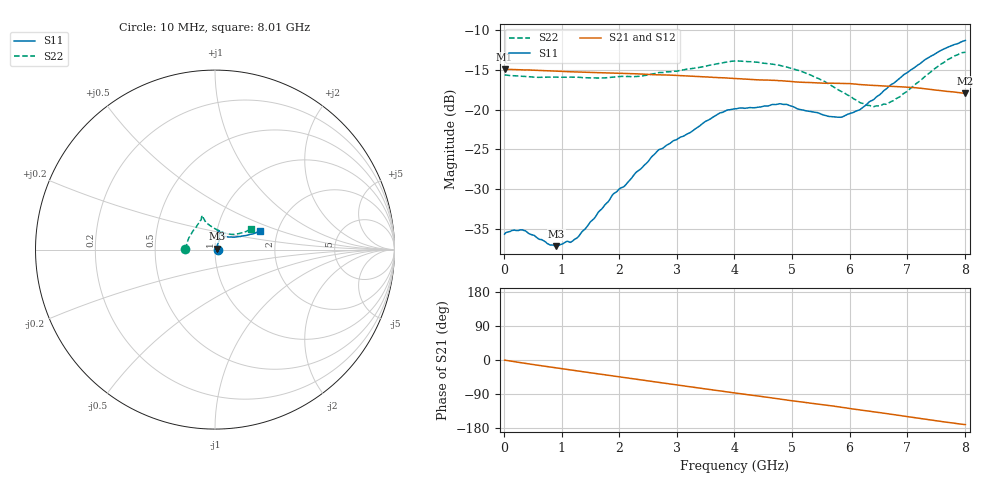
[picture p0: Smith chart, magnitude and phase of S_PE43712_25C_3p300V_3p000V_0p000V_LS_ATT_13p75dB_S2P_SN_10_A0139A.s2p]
! DEVICE ID: PE43712
! File Path: z:\PE43713\PE43713_CHAR_NOM_04292014\AMB\3p300\LS_ATT_13p75dB\PE43713_AMB_3p300V_3p000V_0p000V_LS_ATT_13p75dB_S2P_SN_10_A0139A.s2p
! Serial: 10
! Lot: A0139A
! Temp: 25C
! VDD: 3.300
! VSS: 0.000
! Control_Hi: 3.000
! Control_Lo: 0.000
! Attenuation Step: 13.75dB
! Port 1: RF1
! Port 2: RF2
! ThroughPath:1-2
! IDD: 0.0001471566
! ISS: -7.97e-008
#  Hz  S  RI  R  50
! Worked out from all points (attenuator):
!   801 points, 10 MHz to 8.01 GHz, reference 50 ohm
!   highest |S21| = -14.95 dB at 10 MHz (marker M1); lowest = -18.0 dB at 8.01 GHz (marker M2)
!   lowest |S11| = -37.2 dB at 910 MHz (marker M3), VSWR 1.03, Z = 51.3 + j0.588 ohm
!   |S11| at or under -10 dB: start of sweep to end of sweep
!   |S22| runs from -19.6 to -12.8 dB; largest |S21 - S12| = 0.00065
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1e7  0.0165 0.000311  0.1788 -0.00096  0.179 -0.000902  -0.1649 0.0011
3.3e8  0.0175 0.000531  0.1757 -0.0246  0.1755 -0.0244  -0.1605 0.019
7.8e8  0.0136 0.0041  0.1662 -0.0545  0.1663 -0.0546  -0.1542 0.0424
9.1e8  0.0126 0.00573  0.1625 -0.0625  0.1626 -0.0626  -0.1521 0.0487
1.18e9  0.0108 0.0101  0.1539 -0.0778  0.1539 -0.0779  -0.1468 0.0627
1.35e9  0.0111 0.0129  0.148 -0.0871  0.148 -0.0871  -0.1425 0.07
1.9e9  0.0135 0.0263  0.1254 -0.1137  0.1254 -0.1136  -0.1256 0.0991
2.11e9  0.0147 0.0302  0.1155 -0.1225  0.1155 -0.1224  -0.12 0.1077
2.68e9  0.023 0.0507  0.0856 -0.1411  0.0855 -0.1412  -0.096 0.1408
3.72e9  0.0238 0.0908  0.025 -0.1566  0.0249 -0.1566  -0.0746 0.1793
4.01e9  0.0225 0.0986  0.00817 -0.1565  0.00816 -0.1564  -0.0751 0.1869
4.79e9  0.0206 0.1068  -0.0342 -0.1478  -0.0342 -0.1479  -0.0657 0.1775
5.35e9  0.0309 0.0916  -0.0607 -0.1344  -0.0607 -0.1343  -0.0529 0.1542
5.64e9  0.041 0.0807  -0.073 -0.1268  -0.0729 -0.1268  -0.0357 0.1397
5.88e9  0.0515 0.0739  -0.084 -0.1192  -0.0838 -0.1192  -0.0175 0.1276
6.17e9  0.0704 0.0703  -0.0954 -0.1072  -0.0951 -0.1073  0.00952 0.1107
6.38e9  0.0889 0.0707  -0.1017 -0.0987  -0.1016 -0.0987  0.0318 0.0999
6.68e9  0.1201 0.0709  -0.1106 -0.0857  -0.1104 -0.0858  0.0662 0.0878
6.99e9  0.1517 0.0758  -0.1185 -0.0711  -0.1183 -0.071  0.0977 0.0847
7.37e9  0.1944 0.0846  -0.1241 -0.051  -0.1239 -0.0511  0.1406 0.0916
7.72e9  0.229 0.0941  -0.1252 -0.0339  -0.1251 -0.0339  0.1794 0.104
8.01e9  0.2501 0.1053  -0.1243 -0.021  -0.1241 -0.0212  0.1996 0.1123
